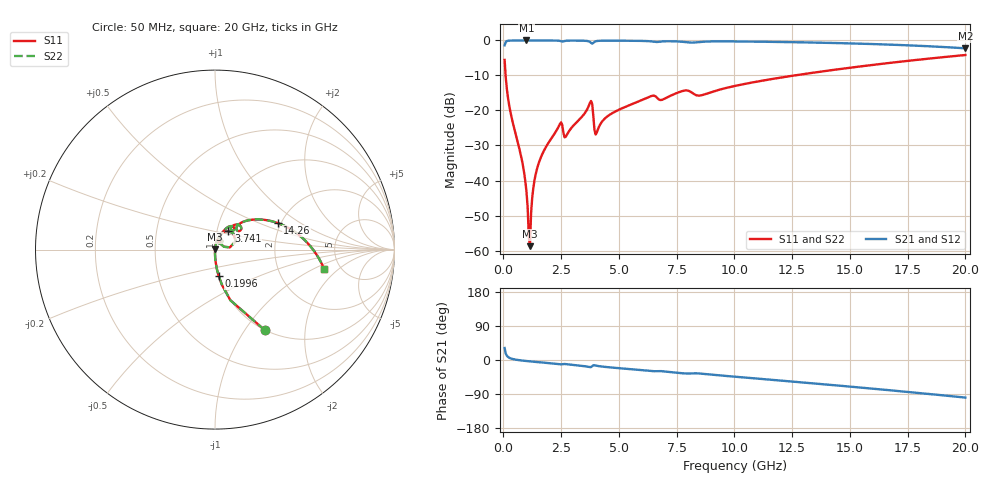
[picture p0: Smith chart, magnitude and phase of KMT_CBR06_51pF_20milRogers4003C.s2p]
! Data measured by Modelithics Inc. support@modelithics.com 813-866-6335
! KEMET CBR0603 51pF, Pad Width= 0.851mm, Pad Length= 0.64mm, Pad Gap= 0.62mm, 20mil Rogers 4003C substrate Data, January 2022
# hz S ma R 50
! 2 Port Network Data from SP1.SP block
! freq  magS11  angS11  magS21  angS21  magS12  angS12  magS22  angS22
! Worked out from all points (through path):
!   401 points, 50 MHz to 20 GHz, reference 50 ohm
!   highest |S21| = -0.01 dB at 997.6 MHz (marker M1); lowest = -2.2 dB at 20 GHz (marker M2)
!   group delay of S21, straight-line fit = 13.9 ps
!   lowest |S11| = -58.8 dB at 1.147 GHz (marker M3), VSWR 1.00, Z = 50.1 + j0.0961 ohm
!   |S11| at or under -10 dB: 93.87 MHz to 12.6 GHz (12.51 GHz wide, 197 % of centre)
!   |S22| runs from -58.8 to -4.2 dB; largest |S21 - S12| = 0
!   S11 on the Smith chart (normalised r, x): 50 MHz: 1.00, -1.24; 199.6 MHz: 1.00, -0.30; 3.741 GHz: 1.13, +0.24; 14.26 GHz: 1.92, +0.66; 20 GHz: 3.74, -1.34
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5e7  0.5269 -58.3  0.8495 31.6  0.8495 31.6  0.5269 -58.3
1.99625e8  0.1491 -81.9  0.9885 7.9  0.9885 7.9  0.1491 -81.9
8.48e8  0.01606 -90.0  0.9993 -1.8  0.9993 -1.8  0.01606 -90.0
9.97625e8  0.006857 -88.3  0.9994 -2.8  0.9994 -2.8  0.006857 -88.3
1.0475e9  0.004139 -85.4  0.9994 -3.1  0.9994 -3.1  0.004139 -85.4
1.14725e9  0.001155 56.2  0.9994 -3.7  0.9994 -3.7  0.001155 56.2
1.197125e9  0.003451 76.1  0.9994 -4.0  0.9994 -4.0  0.003451 76.1
1.396625e9  0.01231 81.8  0.9992 -5.1  0.9992 -5.1  0.01231 81.8
1.74575e9  0.0264 81.2  0.9988 -7.0  0.9988 -7.0  0.0264 81.2
2.444e9  0.06407 67.5  0.9855 -11.3  0.9855 -11.3  0.06407 67.5
2.74325e9  0.04475 68.4  0.9908 -11.2  0.9908 -11.2  0.04475 68.4
3.391625e9  0.08092 71.7  0.9924 -15.3  0.9924 -15.3  0.08092 71.7
3.74075e9  0.1273 54.2  0.955 -18.7  0.955 -18.7  0.1273 54.2
4.04e9  0.04836 52.5  0.9806 -15.3  0.9806 -15.3  0.04836 52.5
4.887875e9  0.09835 67.3  0.9921 -21.0  0.9921 -21.0  0.09835 67.3
6.384125e9  0.1598 55.0  0.9706 -29.1  0.9706 -29.1  0.1598 55.0
6.73325e9  0.1432 47.1  0.9557 -29.1  0.9557 -29.1  0.1432 47.1
1.0025e10  0.2241 44.2  0.9676 -44.1  0.9676 -44.1  0.2241 44.2
1.336662e10  0.3445 27.8  0.9337 -61.4  0.9337 -61.4  0.3445 27.8
1.426438e10  0.3787 23.1  0.9202 -66.2  0.9202 -66.2  0.3787 23.1
1.670825e10  0.4772 9.5  0.8719 -79.7  0.8719 -79.7  0.4772 9.5
2e10  0.6192 -10.3  0.7719 -99.2  0.7719 -99.2  0.6192 -10.3
